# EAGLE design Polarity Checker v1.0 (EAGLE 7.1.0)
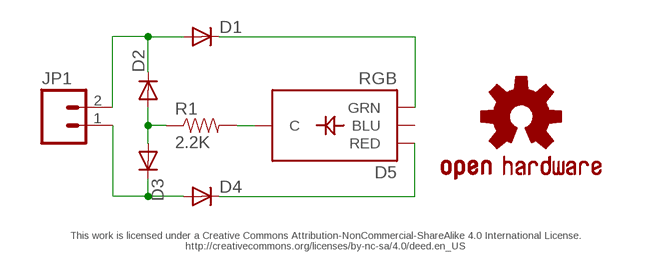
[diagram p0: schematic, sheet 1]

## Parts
D1  DIODE  [DIODE-1N4001-KIT]
D2  DIODE  [DIODE-1N4001-KIT]
D3  DIODE  [DIODE-1N4001-KIT]
D4  DIODE  [DIODE-1N4001-KIT]
D5  RGB  LED-TRICOLOR-THROUGHHOLE  [LED-TRICOLOR-THROUGHHOLE]
JP1  M02JST-PTH-2  [JST-2-PTH]
LOGO1  OSHW-LOGOS  [OSHW-LOGO-S]
R1  2.2K  RESISTORPTH-1/4W  [AXIAL-0.4]

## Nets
N$1: D1.A D2.C JP1.2
N$2: D1.C D5.GRN
N$3: D5.GND(C) R1.P$2
N$4: D2.A D3.A R1.P$1
N$5: D4.C D5.RED
N$6: D3.C D4.A JP1.1
Unconnected: D5.BLU

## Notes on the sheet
- This work is licensed under a Creative Commons Attribution-NonCommercial-ShareAlike 4.0 International License.
  http://creativecommons.org/licenses/by-nc-sa/4.0/deed.en_US

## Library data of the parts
D1-D4 = SparkFun-DiscreteSemi:DIODE: Diode
D5 = E-Paper Display 2:LED-TRICOLOR-THROUGHHOLE
JP1 = SparkFun-Connectors:M02: Standard 2-pin 0.1" header. Use with; PROD_ID: CONN-09863; SKU: PRT-09914
LOGO1 = SparkFun-Aesthetics:OSHW-LOGO: Open Source Hardware Logo
R1 = SparkFun-Resistors:RESISTOR: Resistor

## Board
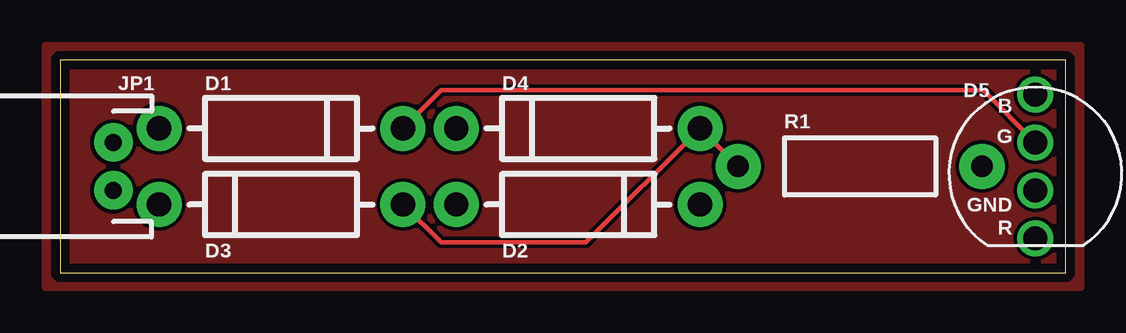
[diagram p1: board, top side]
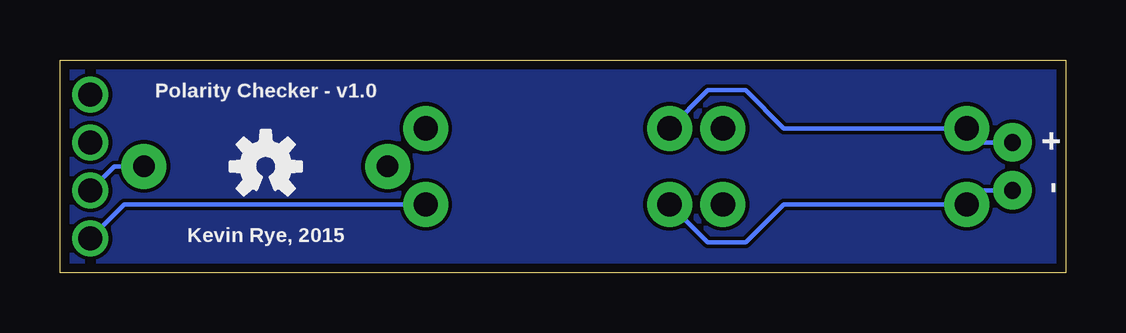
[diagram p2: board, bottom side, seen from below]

Size 41.91 x 8.89 mm. Coordinates in mm from the lower left corner, seen from the top.
Outline: 0,0 41.91,0 41.91,8.89 0,8.89 0,0
Copper layers (1*16): Top 0.0356mm / dielectric 1.5011mm / Bottom 0.0356mm
Design rules "LaenPCBOrder": minimum track width 6mil, minimum drill 13mil, track to track 6mil, track to pad 6mil, pad to pad 6mil, via to via 6mil, smd to smd 6mil, copper to edge 15mil, drill to drill 6mil, minimum pad ring 7mil, minimum via ring 7mil, stop-mask expansion 3mil, vias tented up to drill 0mil, thermal gap 10mil

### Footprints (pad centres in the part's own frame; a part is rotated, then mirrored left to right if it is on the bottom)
DIODE-1N4001-KIT = drill 1.016 pad 1.88: A -5.08,0; C 5.08,0
LED-TRICOLOR-THROUGHHOLE = drill 1: BLU 3,0; GND -1,0; GRN 1,0; RED -3,0
JST-2-PTH = drill 0.7 pad 1.6: 1 -1,0; 2 1,0
AXIAL-0.4 = drill 0.9 pad 1.88: P$1 -5.08,0; P$2 5.08,0

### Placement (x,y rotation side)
D1  9.21,6.03 0 top
D2  21.59,6.03 180 top
D3  9.21,2.86 180 top
D4  21.59,2.86 0 top
D5  40.64,4.45 90 top
JP1  2.22,4.45 90 top
LOGO1  33.34,4.45 0 bottom
R1  33.34,4.45 0 top

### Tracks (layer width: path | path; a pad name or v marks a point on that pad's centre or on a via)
GND
  pour Top: -0.64,9.53 42.55,9.53 42.55,-0.64 -0.64,-0.64
  pour Bottom: -0.32,9.21 42.23,9.21 42.23,-0.32 -0.32,-0.32
N$1
  Bottom 0.178: JP1.2 3.54,5.45 D1.A 11.75,6.03 13.33,7.62 14.92,7.62 D2.C
N$2
  Top 0.178: D1.C 15.88,7.62 38.46,7.62 D5.GRN
N$3
  Bottom 0.178: R1.P$2 39.64,4.45 D5.GND
N$4
  Top 0.178: D3.A 15.88,1.27 21.91,1.27 D2.A R1.P$1
N$5
  Bottom 0.178: D4.C 39.23,2.86 D5.RED
N$6
  Bottom 0.178: JP1.1 3.54,3.44 D3.C 11.75,2.86 13.33,1.27 14.92,1.27 D4.A

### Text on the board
Unrouted: This work is licensed under a Creative Commons Attribution-NonCommercial-ShareAlike 4.0 International License. / http://creativecommons.org/licenses/by-nc-sa/4.0/deed.en_US
tPlace: B | G | GND | R
bNames: Polarity Checker - v1.0 | + | - | Kevin Rye, 2015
